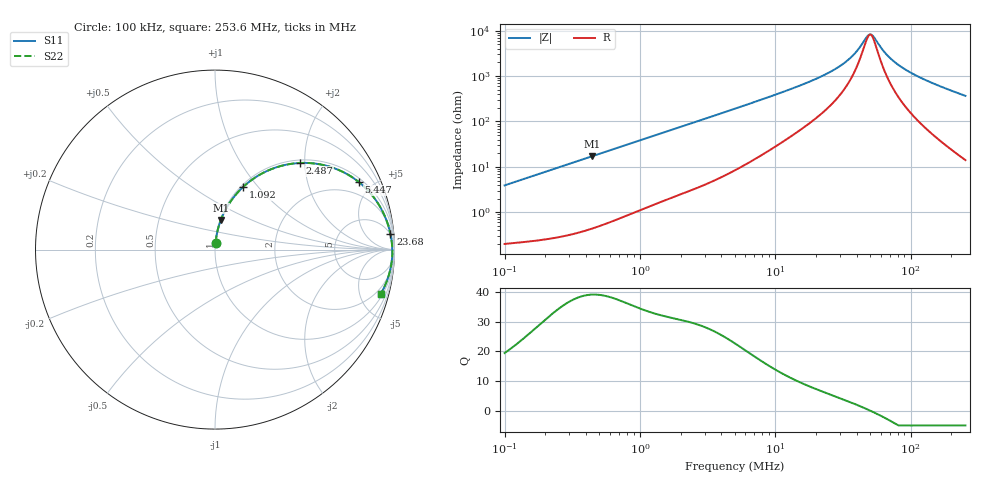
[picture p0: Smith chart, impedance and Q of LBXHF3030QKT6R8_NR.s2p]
! LBXHF3030QKT6R8_NR  S-PARAMETER MODEL  ( General Type )
! Model Generated by TAIYO YUDEN Corporation (http://www.ty-top.com)
! Version 1.0
! TAIYO YUDEN Control No. 210113NI43SB-FBB
! Copyright(c) 2021 TAIYO YUDEN CO.,LTD. All Rights Reserved.
! Product Description (link to TY-COMPAS)
! https://ds.yuden.co.jp/TYCOMPAS/or/detail?pn=LBXHF3030QKT6R8MNR&u=M
! Products Name : Inductors
! Characteristics :
!  Inductance : 6.8 uH , SRF(min) : 35 MHz , DC Resistance(max) : 0.168 Ohm
!  Rated Current : Saturation :900 mA , Temp Rise : 850 mA
!  Case Size : 3.0 x 3.0 / 0.118 x 0.118 [mm/inch] , Thickness : 1.5 / 0.059 [mm/inch]
!  (Conditions: Temperature = 25 degC , DC Bias Current/Voltage = 0A / 0V)
! External Node Assignments :
!  1  o---GGG---o  2
! GND o---------o GND
! Frequency Range : 0.1MHz  -  253.640152MHz  [ 402 STEP ]
# MHz S RI R 50
! Freq[MHz].  S11 Real  S11 Imag  S21 Real  S21 Imag  S12 Real  S12 Imag  S22 Real  S22 Imag
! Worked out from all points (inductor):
!   401 points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, 100 kHz to 253.6 MHz, reference 50 ohm
!   read as one part in series: L = 6.23 uH near 104 kHz
!   highest Q = 39.1 at 443.4 kHz (marker M1), where L = 6.18 uH
!   self-resonance near 49.87 MHz
!   S11 on the Smith chart (normalised r, x): 100 kHz: 1.00, +0.08; 1.092 MHz: 1.02, +0.84; 2.487 MHz: 1.06, +1.89; 5.447 MHz: 1.19, +4.14; 23.68 MHz: 5, +22; 253.6 MHz: 1.28, -7.31
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0.1  0.00355 0.039  0.9965 -0.039  0.9965 -0.039  0.00355 0.039
0.371712  0.024 0.1405  0.976 -0.1405  0.976 -0.1405  0.024 0.1405
0.443406  0.0328 0.1658  0.9672 -0.1658  0.9672 -0.1658  0.0328 0.1658
1.092161  0.1569 0.3492  0.8431 -0.3492  0.8431 -0.3492  0.1569 0.3492
1.381698  0.2255 0.4027  0.7745 -0.4027  0.7745 -0.4027  0.2255 0.4027
2.487307  0.4723 0.4826  0.5277 -0.4826  0.5277 -0.4826  0.4723 0.4826
3.470633  0.6291 0.4648  0.3709 -0.4648  0.3709 -0.4648  0.6291 0.4648
5.03627  0.7752 0.3959  0.2248 -0.3959  0.2248 -0.3959  0.7752 0.3959
5.446922  0.7999 0.3776  0.2001 -0.3776  0.2001 -0.3776  0.7999 0.3776
9.245617  0.9128 0.2503  0.0872 -0.2503  0.0872 -0.2503  0.9128 0.2503
18.72042  0.9696 0.119  0.0304 -0.119  0.0304 -0.119  0.9696 0.119
23.68329  0.9776 0.0863  0.0224 -0.0863  0.0224 -0.0863  0.9776 0.0863
35.04717  0.9853 0.0392  0.0147 -0.0392  0.0147 -0.0392  0.9853 0.0392
40.20007  0.9867 0.024  0.0133 -0.024  0.0133 -0.024  0.9867 0.024
47.02309  0.9878 0.00702  0.0122 -0.00702  0.0122 -0.00702  0.9878 0.00702
49.87039  0.988 0.000652  0.012 -0.000652  0.012 -0.000652  0.988 0.000652
52.8901  0.9881 -0.00573  0.0119 0.00573  0.0119 0.00573  0.9881 -0.00573
61.86696  0.988 -0.023  0.012 0.023  0.012 0.023  0.988 -0.023
69.58603  0.9874 -0.0363  0.0126 0.0363  0.0126 0.0363  0.9874 -0.0363
84.6501  0.9854 -0.0597  0.0146 0.0597  0.0146 0.0597  0.9854 -0.0597
111.3718  0.9799 -0.0962  0.0201 0.0962  0.0201 0.0962  0.9799 -0.0962
253.6402  0.9222 -0.2492  0.0778 0.2492  0.0778 0.2492  0.9222 -0.2492
